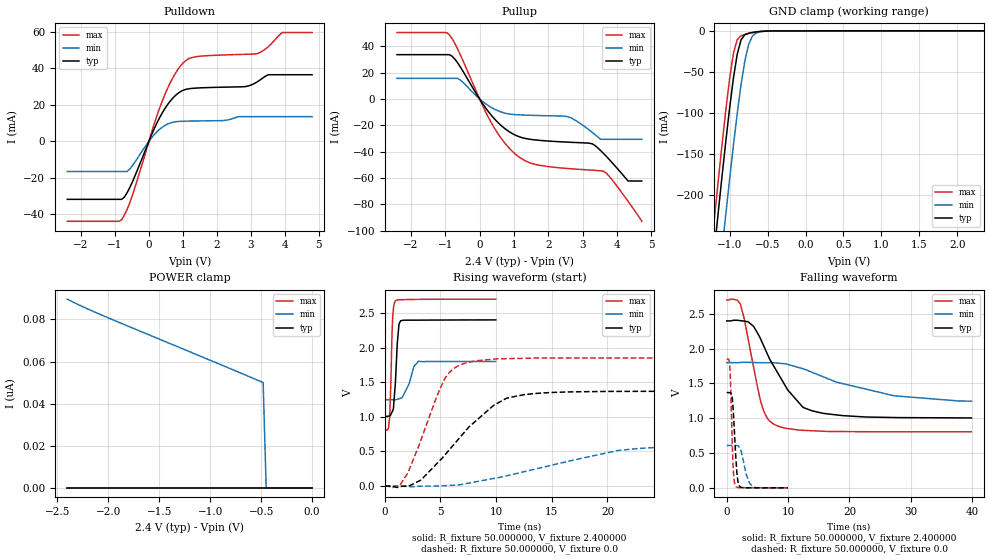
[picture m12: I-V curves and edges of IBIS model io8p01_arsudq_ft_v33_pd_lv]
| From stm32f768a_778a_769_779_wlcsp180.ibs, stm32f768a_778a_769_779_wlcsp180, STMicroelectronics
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|   Model io8p01_arsudq_ft_v33_pd_lv
[Model]  io8p01_arsudq_ft_v33_pd_lv
Model_type I/O
Polarity   Non-Inverting
Enable   Active-Low
Vinl =   0.720000V
Vinh =   1.680000V
Vmeas =  1.200000V
Cref =   50.000000pF
Rref =   100.000000M
Vref =   0.0V
C_comp   2.238700pF   2.180600pF   2.332300pF
[Temperature Range]   25.000000   0.125000k   -40.000000
[Pullup Reference]   2.400000V   1.800000V   2.700000V
[Pulldown Reference]   0.0V   0.0V   0.0V
[POWER Clamp Reference]   2.400000V   1.800000V   2.700000V
[GND Clamp Reference]   0.0V   0.0V   0.0V
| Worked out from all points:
|   slope of the pulldown table from 0 to 0.36 V, typ, clamps not added: 25 ohm
|   slope of the pullup table from 0 to 0.36 V, typ, clamps not added: 27.7 ohm
|   GND clamp passes 1 mA (typ) near -0.62 V on its own axis
|   rising waveform, R_fixture 50.000000, V_fixture 2.400000: 20-80 % time 303ps typ, 741ps min, 199ps max; typ from 1 V to 2.4 V
|   rising waveform, R_fixture 50.000000, V_fixture 0.0: 20-80 % time 4.9ns typ, 9.96ns min, 2.66ns max; typ from 0 V to 1.37 V
|   falling waveform, R_fixture 50.000000, V_fixture 2.400000: 20-80 % time 5.54ns typ, 12.6ns min, 2.64ns max; typ from 2.4 V to 1 V
|   falling waveform, R_fixture 50.000000, V_fixture 0.0: 20-80 % time 534ps typ, 1.03ns min, 386ps max; typ from 1.37 V to 0 V
[Pulldown]
|Voltage   I(typ)   I(min)   I(max)
-2.4V     -31.73mA   -16.51mA   -43.74mA
-800mV    -31.73mA   -16.51mA   -42.87mA
-480mV    -21.98mA   -13.17mA   -29.2mA
80mV      3.63mA     1.966mA    5.014mA
480mV     18.15mA    8.738mA    26.02mA
800mV     25.38mA    10.72mA    37.77mA
1.12V     28.53mA    11.02mA    44.6mA
2.8V      29.84mA    13.47mA    47.53mA
3.2V      32.64mA    13.47mA    48.04mA
3.52V     36.39mA    13.47mA    51.82mA
3.92V     36.39mA    13.47mA    59.43mA
4.8V      36.39mA    13.47mA    59.43mA
[Pullup]
|Voltage   I(typ)   I(min)   I(max)
-2.4V     33.55mA    15.56mA    50.34mA
-960mV    33.55mA    15.56mA    50.34mA
-800mV    32.44mA    15.56mA    45.79mA
-560mV    24.29mA    14.3mA     33.54mA
320mV     -11.75mA   -6.207mA   -17.08mA
960mV     -26.47mA   -11.82mA   -40.02mA
1.52V     -30.88mA   -12.51mA   -49.05mA
2.56V     -32.88mA   -13.48mA   -52.9mA
3.28V     -34.19mA   -25.5mA    -54.18mA
3.6V      -41.31mA   -30.74mA   -54.97mA
4.32V     -62.39mA   -30.74mA   -77.8mA
4.72V     -62.39mA   -30.74mA   -93mA
[GND_clamp]
|Voltage   I(typ)   I(min)   I(max)
-2.4V     -1.424A    -1.508A    -1.394A
-1.25V    -311.2mA   -401.9mA   -273.3mA
-1.2V     -265.4mA   -356.1mA   -227.2mA
-1.15V    -220.4mA   -310.8mA   -181.9mA
-1.1V     -176.3mA   -266.2mA   -137.9mA
-1.05V    -133.8mA   -222.5mA   -95.87mA
-950mV    -57.3mA    -138.9mA   -26.99mA
-900mV    -28.28mA   -100.4mA   -10.6mA
-850mV    -11.02mA   -65.54mA   -5.972mA
-750mV    -2.846mA   -16.51mA   -3.192mA
-600mV    -761.3uA   -1.173mA   -751.9uA
2.35V     58.09uA    37.92uA    67.25uA
[POWER_clamp]
|Voltage   I(typ)   I(min)   I(max)
-2.4V     0A         89.62nA    0A
-2.04V    0A         81.57nA    0A
-480mV    0A         50.01nA    0A
-450mV    0A         0A         0A
0V        0A         0A         0A
[Ramp]
| variable   typ   min   max
dV/dt_r  0.82164/4.89960n   0.36428/9.97952n   1.11030/2.65333n
dV/dt_f  0.83736/5.55236n   0.32262/12.66971n   1.13705/2.64083n
R_load = 50.000000
[Rising Waveform]
R_fixture= 50.000000
V_fixture= 2.400000
V_fixture_min= 1.800000
V_fixture_max= 2.700000
|time   V(typ)   V(min)   V(max)
0s        1.005V     1.245V     804.5mV
320.3ps   1.01V      1.245V     822.6mV
440.4ps   1.015V     1.245V     997.9mV
720.7ps   1.094V     1.245V     2.46V
961ps     1.513V     1.245V     2.672V
1.121ns   2.054V     1.253V     2.687V
1.281ns   2.34V      1.261V     2.69V
1.421ns   2.386V     1.268V     2.691V
3.023ns   2.395V     1.802V     2.695V
9.97ns    2.399V     1.799V     2.699V
[Rising Waveform]
R_fixture= 50.000000
V_fixture= 0.0
V_fixture_min= 0.0
V_fixture_max= 0.0
|time   V(typ)   V(min)   V(max)
0s        85.33uV    35.72uV    197.6uV
1.361ns   -8.665mV   -381.4uV   17.59mV
2.002ns   2.242mV    -5.156mV   171.2mV
3.283ns   93.39mV    -541uV     679.2mV
5.365ns   442.8mV    5.672mV    1.542V
7.207ns   788mV      33.22mV    1.774V
9.77ns    1.164V     109.4mV    1.832V
12.89ns   1.326V     221.9mV    1.846V
22.74ns   1.367V     542.4mV    1.85V
39.88ns   1.369V     608.5mV    1.85V
[Falling Waveform]
R_fixture= 50.000000
V_fixture= 2.400000
V_fixture_min= 1.800000
V_fixture_max= 2.700000
|time   V(typ)   V(min)   V(max)
0s        2.399V     1.799V     2.699V
2.242ns   2.402V     1.801V     2.637V
4.324ns   2.324V     1.802V     1.758V
5.606ns   2.123V     1.799V     1.22V
6.567ns   1.933V     1.798V     1.009V
7.688ns   1.745V     1.798V     914.5mV
9.93ns    1.408V     1.775V     851.8mV
13.85ns   1.108V     1.662V     820.9mV
27.31ns   1.011V     1.323V     804.7mV
39.88ns   1.005V     1.245V     804.5mV
[Falling Waveform]
R_fixture= 50.000000
V_fixture= 0.0
V_fixture_min= 0.0
V_fixture_max= 0.0
|time   V(typ)   V(min)   V(max)
0s        1.369V     608.5mV    1.85V
460.5ps   1.37V      608.3mV    1.789V
660.7ps   1.365V     608.2mV    1.397V
1.041ns   1.144V     607.9mV    308.8mV
1.421ns   520.8mV    608.8mV    29.01mV
1.802ns   105.6mV    605.6mV    5.422mV
2.202ns   13.05mV    564.4mV    2.46mV
3.143ns   1.285mV    199.1mV    1.509mV
4.364ns   793.3uV    8.303mV    945.5uV
9.97ns    85.33uV    35.72uV    197.6uV
